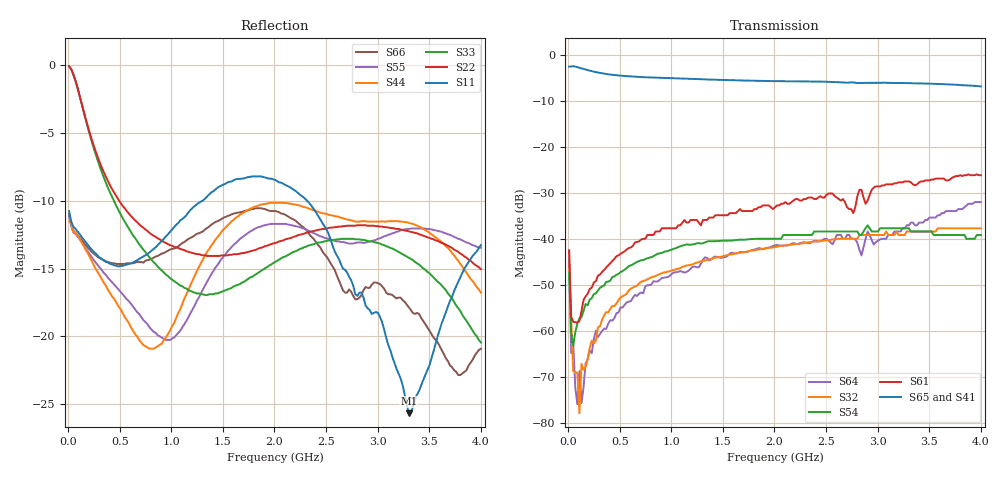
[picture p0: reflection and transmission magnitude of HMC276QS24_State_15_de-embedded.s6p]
! Hittite Microwave Corporation
! 20 Alpha Road
! Chelmsford, MA 01824
! Tel: 978-250-3343
! Fax: 978-250-3373
! Device: HMC276QS24, 0.7-3.0 GHz, GaAS MMIC 4x2 Switch Matrix in 24-lead QSOP package
! Misc: Data was de-embedded to package pins.
!  Port 1 = OP1
!  Port 2 = VL
!  Port 3 = VH
!  Port 4 = HH
!  Port 5 = HL
!  Port 6 = OP2
!  Vdd = +5 V
!  Vctl = 0 V[Logic 0] / +5 V[Logic 1]
!  State 15,  HH to OP1,  HL to OP2
!  Control Lines (Logic)
!  HV 1 = 1, Tone 1 = 1
!  HV 2 = 1, Tone 2 = 0
!  Data reformated to new Touchstone file format - Wed Jan 10 16:00:54 2007
# MHz S DB R 50
! 6 Port Network Data
! freq  dbS11  angS11  dbS12  angS12  dbS13  angS13  dbS14  angS14
!  dbS15  angS15  dbS16  angS16
!  dbS21  angS21  dbS22  angS22
!  dbS23  angS23  dbS24  angS24  dbS25  angS25  dbS26  angS26
!  dbS31  angS31  dbS32  angS32  dbS33  angS33  dbS34  angS34
!  dbS35  angS35  dbS36  angS36
!  dbS41  angS41  dbS42  angS42
!  dbS43  angS43  dbS44  angS44  dbS45  angS45  dbS46  angS46
!  dbS51  angS51  dbS52  angS52  dbS53  angS53  dbS54  angS54
!  dbS55  angS55  dbS56  angS56
!  dbS61  angS61  dbS62  angS62
!  dbS63  angS63  dbS64  angS64  dbS65  angS65  dbS66  angS66
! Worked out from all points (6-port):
!   201 points, 10 MHz to 4 GHz, reference 50 ohm
!   strongest paths, dB at 10 MHz, 1.008 GHz, 2.005 GHz, 3.002 GHz, 4 GHz:
!     S65: -2.6, -5.1, -5.8, -6.1, -6.9
!     S41: -2.8, -5.3, -6.1, -6.2, -6.9
!     S61: -42.6, -37.7, -33.2, -28.6, -26.2
!     S54: -47.4, -42.3, -40.0, -38.4, -39.2
!     S32: -45.3, -46.9, -41.8, -39.2, -37.7
!     S64: -42.5, -47.6, -41.4, -40.4, -32.0
!   lowest |S11| = -25.7 dB at 3.302 GHz (marker M1), VSWR 1.11, Z = 54.3 + j3.36 ohm
!   |S11| at or under -10 dB: start of sweep to 1.302 GHz; 2.317 GHz to end of sweep
